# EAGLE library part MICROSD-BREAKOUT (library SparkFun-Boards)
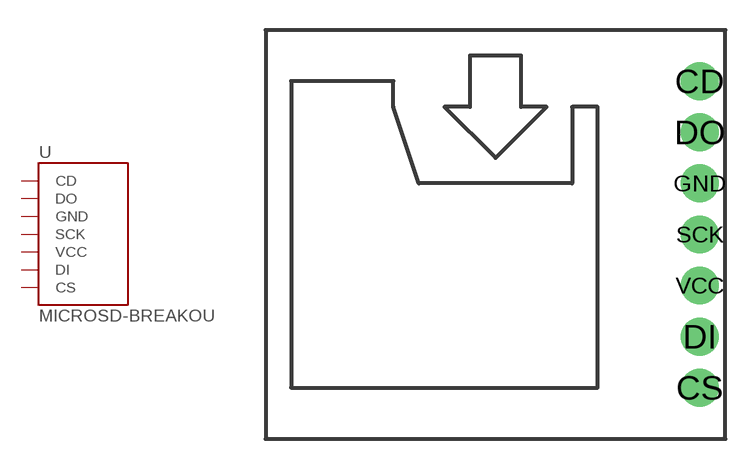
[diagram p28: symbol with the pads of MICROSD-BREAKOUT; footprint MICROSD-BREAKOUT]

Designator prefix U

## MICROSD-BREAKOUT  [MICROSD-BREAKOUT]
CD  CD
CS  CS
DI  DI
DO  DO
GND  GND  pwr
SCK  SCK
VCC  VCC

## Footprint MICROSD-BREAKOUT (pad centres in mm)
drill 1.118 pad 1.88: CD 12.7,8.89; CS 12.7,-6.35; DI 12.7,-3.81; DO 12.7,6.35; GND 12.7,3.81; SCK 12.7,1.27; VCC 12.7,-1.27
